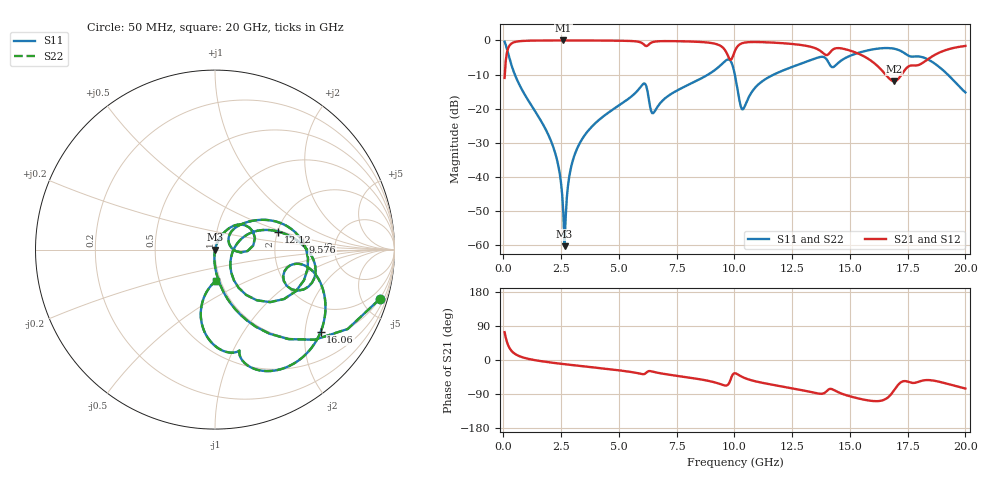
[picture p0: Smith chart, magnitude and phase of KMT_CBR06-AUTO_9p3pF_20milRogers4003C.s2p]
! Data measured by Modelithics Inc. support@modelithics.com 813-866-6335
! KEMET CBR06-AUTO 9.3pF, Pad Width= 0.851mm, Pad Length= 0.64mm, Pad Gap= 0.62mm, 20mil Rogers 4003C substrate Data, January 2022
# hz S ma R 50
! 2 Port Network Data from SP1.SP block
! freq  magS11  angS11  magS21  angS21  magS12  angS12  magS22  angS22
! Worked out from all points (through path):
!   401 points, 50 MHz to 20 GHz, reference 50 ohm
!   highest |S21| = -0.01 dB at 2.594 GHz (marker M1); lowest = -12.0 dB at 16.91 GHz (marker M2)
!   group delay of S21, straight-line fit = 13.2 ps
!   lowest |S11| = -60.3 dB at 2.643 GHz (marker M3), VSWR 1.00, Z = 50.1 - j0.0375 ohm
!   |S11| at or under -10 dB: 492.9 MHz to 8.861 GHz (8.368 GHz wide, 179 % of centre); 10.02 GHz to 11.7 GHz (1.688 GHz wide, 15.5 % of centre); 19.24 GHz to end of sweep
!   |S22| runs from -60.3 to -0.4 dB; largest |S21 - S12| = 0
!   S11 on the Smith chart (normalised r, x): 50 MHz: 0.98, -6.71; 9.576 GHz: 2.89, +0.33; 12.12 GHz: 2.01, +0.47; 16.06 GHz: 1.17, -2.42; 20 GHz: 0.95, -0.34
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5e7  0.9592 -16.6  0.2823 73.4  0.2823 73.4  0.9592 -16.6
2.99375e8  0.4889 -61.9  0.8718 28.0  0.8718 28.0  0.4889 -61.9
5.4875e8  0.2846 -75.7  0.958 14.2  0.958 14.2  0.2846 -75.7
2.14475e9  0.02818 -95.6  0.9987 -7.4  0.9987 -7.4  0.02818 -95.6
2.394125e9  0.01353 -95.4  0.9989 -9.3  0.9989 -9.3  0.01353 -95.4
2.593625e9  0.002923 -82.0  0.999 -10.7  0.999 -10.7  0.002923 -82.0
2.6435e9  0.000967 -22.8  0.999 -11.1  0.999 -11.1  0.000967 -22.8
2.94275e9  0.01458 72.9  0.9988 -13.2  0.9988 -13.2  0.01458 72.9
3.391625e9  0.03521 72.0  0.9981 -16.2  0.9981 -16.2  0.03521 72.0
6.035e9  0.2279 32.4  0.8982 -37.5  0.8982 -37.5  0.2279 32.4
6.434e9  0.08614 15.4  0.9377 -30.3  0.9377 -30.3  0.08614 15.4
6.73325e9  0.1143 45.4  0.9732 -34.4  0.9732 -34.4  0.1143 45.4
9.576125e9  0.4909 5.1  0.734 -67.2  0.734 -67.2  0.4909 5.1
1.0025e10  0.3065 -55.5  0.707 -34.9  0.707 -34.9  0.3065 -55.5
1.037412e10  0.09808 -10.1  0.9183 -45.7  0.9183 -45.7  0.09808 -10.1
1.211975e10  0.3648 16.0  0.909 -70.5  0.909 -70.5  0.3648 16.0
1.336662e10  0.5243 -1.5  0.7965 -85.3  0.7965 -85.3  0.5243 -1.5
1.605988e10  0.7458 -37.9  0.4627 -108.5  0.4627 -108.5  0.7458 -37.9
1.670825e10  0.7712 -56.0  0.2754 -95.4  0.2754 -95.4  0.7712 -56.0
1.690775e10  0.7567 -62.3  0.252 -80.3  0.252 -80.3  0.7567 -62.3
1.865338e10  0.4626 -97.2  0.6083 -54.7  0.6083 -54.7  0.4626 -97.2
2e10  0.1731 -88.2  0.8299 -75.3  0.8299 -75.3  0.1731 -88.2
